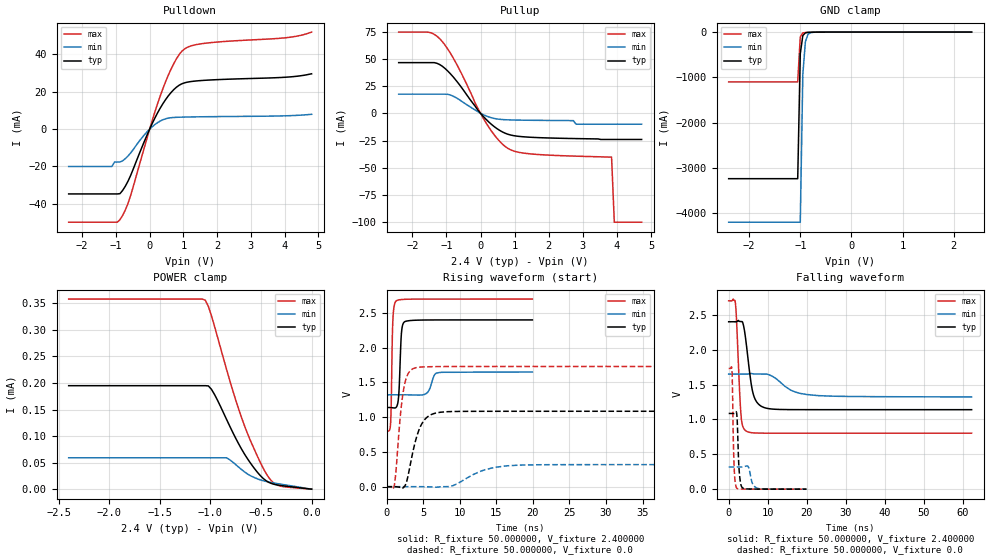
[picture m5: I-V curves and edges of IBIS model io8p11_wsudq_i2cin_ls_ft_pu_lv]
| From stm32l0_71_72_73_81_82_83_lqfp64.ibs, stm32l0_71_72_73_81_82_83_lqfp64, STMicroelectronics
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|   Model io8p11_wsudq_i2cin_ls_ft_pu_lv
[Model]  io8p11_wsudq_i2cin_ls_ft_pu_lv
Model_type I/O
Polarity   Non-Inverting
Enable   Active-Low
Vinl =   0.720000V
Vinh =   1.680000V
Vmeas =  1.200000V
Cref =   50.000000pF
Rref =   100.000000M
Vref =   0.0V
C_comp   2.943600pF   2.919700pF   2.965100pF
[Temperature Range]   25.000000   0.105000k   -40.000000
[Pullup Reference]   2.400000V   1.650000V   2.700000V
[Pulldown Reference]   0.0V   0.0V   0.0V
[POWER Clamp Reference]   2.400000V   1.650000V   2.700000V
[GND Clamp Reference]   0.0V   0.0V   0.0V
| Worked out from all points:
|   slope of the pulldown table from 0 to 0.36 V, typ, clamps not added: 28.5 ohm
|   slope of the pullup table from 0 to 0.36 V, typ, clamps not added: 32.2 ohm
|   GND clamp passes 1 mA (typ) near -0.65 V on its own axis
|   rising waveform, R_fixture 50.000000, V_fixture 2.400000: 20-80 % time 287ps typ, 641ps min, 197ps max; typ from 1.14 V to 2.4 V
|   rising waveform, R_fixture 50.000000, V_fixture 0.0: 20-80 % time 1.59ns typ, 3.84ns min, 929ps max; typ from 0.001 V to 1.09 V
|   falling waveform, R_fixture 50.000000, V_fixture 2.400000: 20-80 % time 1.81ns typ, 5.25ns min, 917ps max; typ from 2.4 V to 1.14 V
|   falling waveform, R_fixture 50.000000, V_fixture 0.0: 20-80 % time 493ps typ, 872ps min, 391ps max; typ from 1.09 V to 0.001 V
[Pulldown]
|Voltage   I(typ)   I(min)   I(max)
-2.4V     -34.7mA    -20mA      -49.82mA
-1.12V    -34.7mA    -20mA      -49.82mA
-1.04V    -34.7mA    -17.61mA   -49.82mA
-880mV    -34.55mA   -17.61mA   -48.46mA
-560mV    -24.65mA   -12.68mA   -35.33mA
0V        0A         0A         0A
400mV     13.84mA    5.066mA    22.03mA
720mV     21.25mA    6.254mA    35.26mA
1.04V     24.83mA    6.464mA    43.02mA
1.6V      26.11mA    6.627mA    45.88mA
4V        27.76mA    7.125mA    48.87mA
4.8V      29.63mA    7.94mA     51.96mA
[Pullup]
|Voltage   I(typ)   I(min)   I(max)
-2.4V     46.57mA    17.6mA     74.62mA
-1.52V    46.57mA    17.6mA     74.51mA
-1.2V     44.84mA    17.6mA     68.64mA
-720mV    30.34mA    14.43mA    46.24mA
-160mV    6.617mA    3.074mA    9.467mA
160mV     -5.477mA   -2.361mA   -8.695mA
480mV     -14.04mA   -5.167mA   -22.91mA
800mV     -19.21mA   -5.978mA   -32.18mA
1.52V     -22.07mA   -6.4mA     -37.42mA
3.84V     -24mA      -10mA      -40.2mA
3.92V     -24mA      -10mA      -100mA
4.72V     -24mA      -10mA      -100mA
[GND_clamp]
|Voltage   I(typ)   I(min)   I(max)
-2.4V     -3.237A    -4.198A    -1.1A
-1.05V    -3.237A    -4.198A    -1.1A
-1V       -475.8mA   -4.198A    -104.2mA
-950mV    -76.24mA   -935.4mA   -18.39mA
-900mV    -16.61mA   -212.9mA   -9.105mA
-850mV    -6.547mA   -50.94mA   -6.589mA
-800mV    -3.998mA   -13.81mA   -4.86mA
-650mV    -1.043mA   -1.182mA   -1.146mA
2.35V     0A         0A         0A
[POWER_clamp]
|Voltage   I(typ)   I(min)   I(max)
-2.4V     195uA      59.14uA    358.2uA
-1.05V    195uA      59.14uA    356uA
-1.02V    194.5uA    59.14uA    344.5uA
-960mV    178.7uA    59.14uA    307.4uA
-840mV    131.4uA    59.14uA    225.5uA
-690mV    74.82uA    36.58uA    133.7uA
-600mV    48.08uA    24.92uA    89.53uA
-510mV    26.23uA    17.69uA    51.64uA
-450mV    15.91uA    14.53uA    29.77uA
-390mV    10.19uA    12.23uA    14.39uA
-330mV    7.608uA    10.24uA    6.963uA
0V        0A         0A         0A
[Ramp]
| variable   typ   min   max
dV/dt_r  0.65095/1.58313n   0.19036/3.83818n   1.03799/0.92484n
dV/dt_f  0.75618/1.80820n   0.19410/5.23041n   1.13779/0.91464n
R_load = 50.000000
[Rising Waveform]
R_fixture= 50.000000
V_fixture= 2.400000
V_fixture_min= 1.650000
V_fixture_max= 2.700000
|time   V(typ)   V(min)   V(max)
0s        1.14V      1.323V     802.6mV
560.6ps   1.139V     1.323V     918.3mV
880.9ps   1.135V     1.323V     2.428V
1.321ns   1.143V     1.323V     2.673V
1.682ns   1.338V     1.323V     2.688V
2.042ns   2.213V     1.323V     2.693V
2.442ns   2.371V     1.323V     2.696V
5.365ns   2.399V     1.337V     2.7V
7.167ns   2.4V       1.642V     2.7V
19.94ns   2.4V       1.65V      2.7V
[Rising Waveform]
R_fixture= 50.000000
V_fixture= 0.0
V_fixture_min= 0.0
V_fixture_max= 0.0
|time   V(typ)   V(min)   V(max)
0s        878.1uV    1.336mV    737.2uV
1.001ns   990.5uV    1.333mV    -10.1mV
1.251ns   187.8uV    1.33mV     175.1mV
2.002ns   -15.72mV   1.327mV    1.139V
2.377ns   -5.02mV    1.343mV    1.424V
4.004ns   675.9mV    1.415mV    1.712V
5.506ns   997mV      -428.3uV   1.726V
8.258ns   1.079V     1.647mV    1.729V
16.52ns   1.086V     301.5mV    1.73V
62.31ns   1.086V     318.6mV    1.73V
[Falling Waveform]
R_fixture= 50.000000
V_fixture= 2.400000
V_fixture_min= 1.650000
V_fixture_max= 2.700000
|time   V(typ)   V(min)   V(max)
0s        2.4V       1.65V      2.7V
1.752ns   2.4V       1.65V      2.657V
3.128ns   2.403V     1.65V      1.09V
3.879ns   2.327V     1.65V      868.8mV
4.63ns    2.029V     1.65V      828.9mV
5.756ns   1.516V     1.658V     810.9mV
6.381ns   1.349V     1.652V     807.4mV
9.384ns   1.165V     1.65V      803.3mV
19.77ns   1.14V      1.359V     802.6mV
62.31ns   1.14V      1.323V     802.6mV
[Falling Waveform]
R_fixture= 50.000000
V_fixture= 0.0
V_fixture_min= 0.0
V_fixture_max= 0.0
|time   V(typ)   V(min)   V(max)
0s        1.086V     318.6mV    1.73V
840.8ps   1.086V     318.6mV    1.711V
1.361ns   1.085V     318.6mV    378.8mV
1.602ns   1.091V     318.6mV    138.5mV
2.042ns   1.091V     318.6mV    18.18mV
2.723ns   245.1mV    318.4mV    4.391mV
3.483ns   23.24mV    318.8mV    2.637mV
4.965ns   3.471mV    325.8mV    1.438mV
7.648ns   1.532mV    8.874mV    911.1uV
19.94ns   878.1uV    1.336mV    737.2uV
